(* Logix 5000 AddOnInstructionDefinition export SB2_Reader; software revision 19.01 *)

ADD_ON_INSTRUCTION SB2_Reader   (* revision 2.3, vendor Jennings Electric Technology *)
VAR_INPUT
   Clock : BOOL; {required}
   Data : BOOL; {required}
END_VAR
VAR_IN_OUT
   Ser_String_Temp : STRING; {required}
   Ser_String : STRING; {required}
   Reading : STRING; {required}
   Disconnected_String : STRING; {required}
END_VAR
VAR
   Serial_Num_Restart : TIMER := (PRE := 750); {access None}
   Read_ONS : BOOL; {access None}
   First_Scan : BOOL; {access None}
   Parity_Fail : BOOL; {access None}
   Ser_Num_Bit_CU : DINT; {access None}
   Ser_Char_Num : DINT; {access None}
   Ser_Clock_ONS : BOOL; {access None}
   AsciiChar : SINT; {access None}
   Parity_SINT : SINT; {access None}
   Parity_BOOL : BOOL; {access None}
   Parity_Fail_CTU : COUNTER := (PRE := 999999); {access None}
   Disconnected : TIMER := (PRE := 1500); {access None}
END_VAR

ROUTINE Logic   (* ladder *)
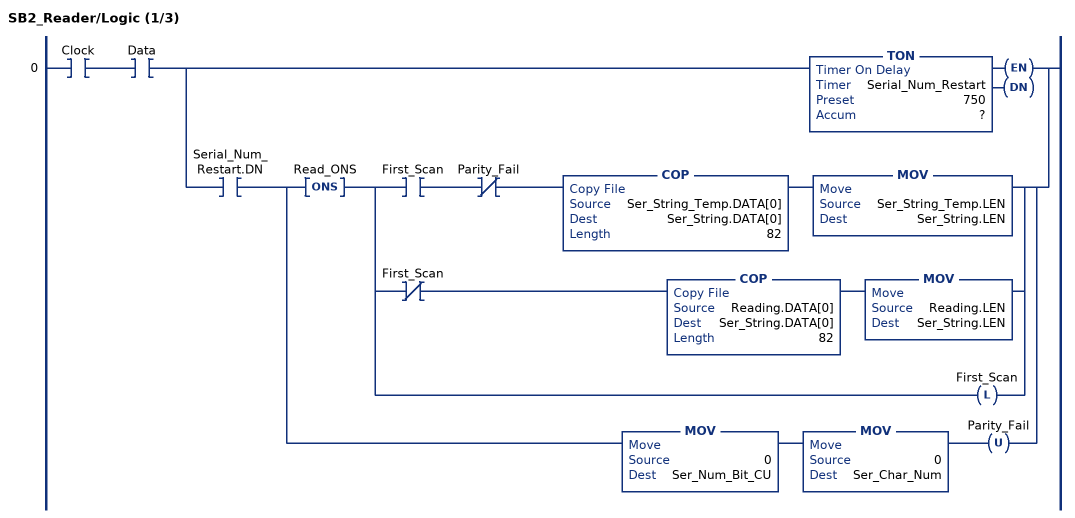
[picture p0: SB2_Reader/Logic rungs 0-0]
   0: XIC(Clock)XIC(Data)[TON(Serial_Num_Restart,?,?) ,XIC(Serial_Num_Restart.DN) [ONS(Read_ONS) [XIC(First_Scan) XIO(Parity_Fail) COP(Ser_String_Temp.DATA[0],Ser_String.DATA[0],82) MOV(Ser_String_Temp.LEN,Ser_String.LEN) ,XIO(First_Scan) COP(Reading.DATA[0],Ser_String.DATA[0],82) MOV(Reading.LEN,Ser_String.LEN) ,OTL(First_Scan) ] ,MOV(0,Ser_Num_Bit_CU) MOV(0,Ser_Char_Num) OTU(Parity_Fail) ] ];
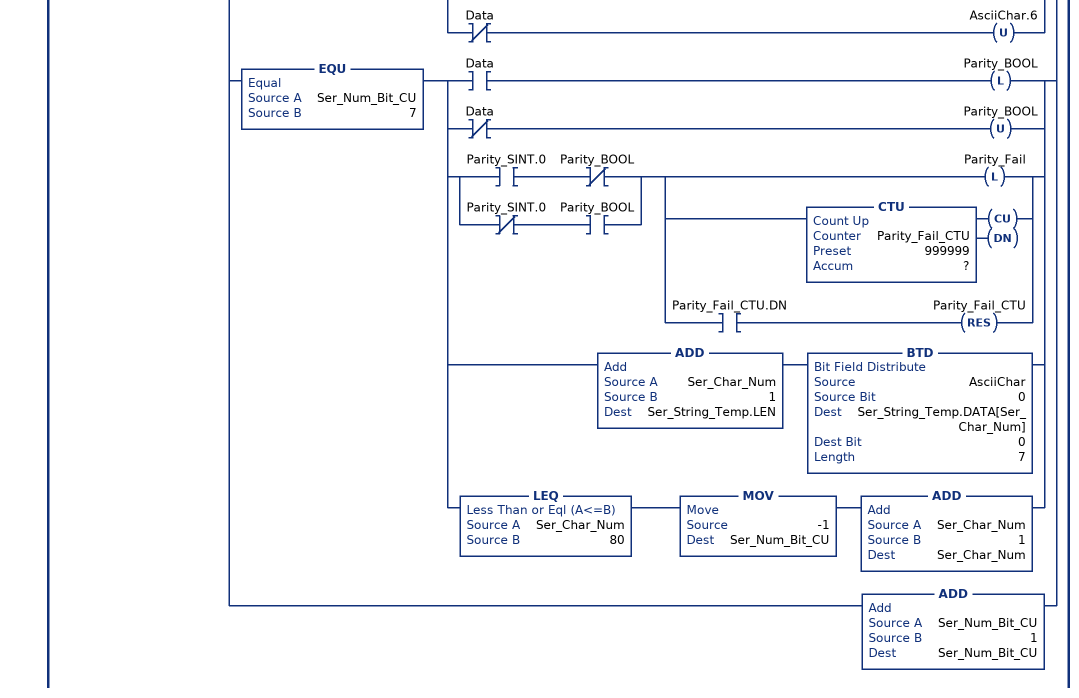
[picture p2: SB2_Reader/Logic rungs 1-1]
   1: XIC(Clock)ONS(Ser_Clock_ONS)[EQU(Ser_Num_Bit_CU,0) [XIC(Data) OTL(AsciiChar.0) MOV(0,Parity_SINT) ,XIO(Data) OTU(AsciiChar.0) MOV(1,Parity_SINT) ] ,EQU(Ser_Num_Bit_CU,1) [XIC(Data) OTL(AsciiChar.1) ADD(Parity_SINT,1,Parity_SINT) ,XIO(Data) OTU(AsciiChar.1) ] ,EQU(Ser_Num_Bit_CU,2) [XIC(Data) OTL(AsciiChar.2) ADD(Parity_SINT,1,Parity_SINT) ,XIO(Data) OTU(AsciiChar.2) ] ,EQU(Ser_Num_Bit_CU,3) [XIC(Data) OTL(AsciiChar.3) ADD(Parity_SINT,1,Parity_SINT) ,XIO(Data) OTU(AsciiChar.3) ] ,EQU(Ser_Num_Bit_CU,4) [XIC(Data) OTL(AsciiChar.4) ADD(Parity_SINT,1,Parity_SINT) ,XIO(Data) OTU(AsciiChar.4) ] ,EQU(Ser_Num_Bit_CU,5) [XIC(Data) OTL(AsciiChar.5) ADD(Parity_SINT,1,Parity_SINT) ,XIO(Data) OTU(AsciiChar.5) ] ,EQU(Ser_Num_Bit_CU,6) [XIC(Data) OTL(AsciiChar.6) ADD(Parity_SINT,1,Parity_SINT) ,XIO(Data) OTU(AsciiChar.6) ] ,EQU(Ser_Num_Bit_CU,7) [XIC(Data) OTL(Parity_BOOL) ,XIO(Data) OTU(Parity_BOOL) ,[XIC(Parity_SINT.0) XIO(Parity_BOOL) ,XIO(Parity_SINT.0) XIC(Parity_BOOL) ] [OTL(Parity_Fail) ,CTU(Parity_Fail_CTU,?,?) ,XIC(Parity_Fail_CTU.DN) RES(Parity_Fail_CTU) ] ,ADD(Ser_Char_Num,1,Ser_String_Temp.LEN) BTD(AsciiChar,0,Ser_String_Temp.DATA[Ser_Char_Num],0,7) ,LEQ(Ser_Char_Num,80) MOV(-1,Ser_Num_Bit_CU) ADD(Ser_Char_Num,1,Ser_Char_Num) ] ,ADD(Ser_Num_Bit_CU,1,Ser_Num_Bit_CU) ];
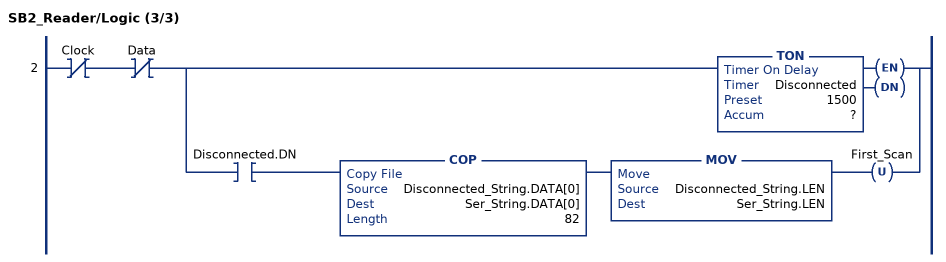
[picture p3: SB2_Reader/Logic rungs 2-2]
   2: XIO(Clock)XIO(Data)[TON(Disconnected,?,?) ,XIC(Disconnected.DN) COP(Disconnected_String.DATA[0],Ser_String.DATA[0],82) MOV(Disconnected_String.LEN,Ser_String.LEN) OTU(First_Scan) ];
END_ROUTINE
END_ADD_ON_INSTRUCTION
